
DATA_BLOCK DB3417
TITLE=
VERSION : 0.1

STRUCT
   CM_ID : STRING  [8 ] := '=PRM'; //COMPOSITE MACHINE
   STATION_ID : STRING  [8 ] := '++OP10'; //STATION - TRATTO - ZONE
   ELEMENT_ID : STRING  [8 ] := '+80FAN95'; //ELEMENT
   DB_ID : INT := 1 ; //DB SIZE OR TYPE
   PART_STYLE : STRING  [12 ]; //PART STYLE ON LAST STATION
   ACT_CYCLE_TIME : INT ; //ACTUAL CYCLE TIME FOR THIS STYLE
   COUNT_GOOD : INT ; //COUNTER GOOD PIECES
   COUNT_SCRAP : INT ; //COUNTER SCRAP PIECES
   SPARE_00 : ARRAY  [0 .. 15 ] OF //SPARE INTEGER
   INT ;
   SPARE_01 : ARRAY  [0 .. 17 ] OF //SPARE INTEGER
   INT ;
   CODE_EVENT : ARRAY  [0 .. 7 ] OF //CODE EVENT - EXTENDED FAULT CODE DIAGNOSTIC
   INT ;
   EVENT : STRUCT
E0000 : BOOL ; //+80FAN95-U1;MS.GENERALI ERRORE;1
E0001 : BOOL ; //+80FAN95-U1;MS.GENERALI AVVERTIMENTO;2
E0002 : BOOL ; //+80FAN95-U1;MS.MODALITA MANUALE;16
E0003 : BOOL ; //+80FAN95-U1;MS.MODO AUTOMATICO;19
E0004 : BOOL ; //+80FAN95-U1;MS.RILASCIO;17
E0005 : BOOL ; //+80FAN95-U1; MS. MOTORE ON;58
E0006 : BOOL ; //+80FAN95-U1; MS. MOTORE OFF;58
E0007 : BOOL ; //+80FAN95-U1; MS. MOTORE ON FRONTE POSITIVO;58
E0008 : BOOL ; //+80FAN95-U1; MS. FREQUENZA OK;58
E0009 : BOOL ; //+80FAN95-U1; MS. LOCALE DI CONTROLLO INTERRUTTORE ABILITATO;58
E0010 : BOOL ; //+80FAN95-U1; MS. ARRESTO A SUO AGIO;58
E0011 : BOOL ; //+80FAN95-U1; MS. LAST TASTO PREMUTO;58
E0012 : BOOL ; //+80FAN95-U1; MS. MS_14;58
E0013 : BOOL ; //+80FAN95-U1; MS. MS_15;58
E0014 : BOOL ; //+80FAN95-U1; MS. RES_WO_SAFETY_TEST;58
E0015 : BOOL ; //+80FAN95-U1; MS. MOTORE OFF FRONTE NEGATIVO;58
E0016 : BOOL ; //+80FAN95-U1;ME.MOTORE PROTEZIONE NON OK;1
E0017 : BOOL ; //+80FAN95-U1;ME.RUNTIME;1
E0018 : BOOL ; //+80FAN95-U1;ME.FREQUENZA CONVERTITORE PRONTO ERRORE;1
E0019 : BOOL ; //+80FAN95-U1;ME.FREQUENZA CONVERTITORE INTERNO ERRORE;1
E0020 : BOOL ; //+80FAN95-U1;ME.FREQUENZA CONVERTITORE DI VELOCITA ERRORE;1
E0021 : BOOL ; //+80FAN95-U1;ME.FREQUENZA CONVERTITORE MOTORE SOVRACCARICO;1
E0022 : BOOL ; //+80FAN95-U1; ME. FREQUENZA CONVERTITORE MOTORE SOVRACCARICO;58
E0023 : BOOL ; //+80FAN95-U1;ME.FREQUENZA CONVERTITORE AVVERTIMENTO;2
E0024 : BOOL ; //+80FAN95-U1; ME. FREQUENZA CONVERTITORE CORRENTE LIMITE DI ATTENZIONE;58
E0025 : BOOL ; //+80FAN95-U1;ME.PTC AVVERTIMENTO;2
E0026 : BOOL ; //+80FAN95-U1;ME.INTERRUTTORE PER MANUTENZIONE ERROR RILASCIO;1
E0027 : BOOL ; //+80FAN95-U1;ME.INTERRUTTORE PER MANUTENZIONE ERROR CORRENTE TAGLIARE;1
E0028 : BOOL ; //+80FAN95-U1; ME. ME_14;58
E0029 : BOOL ; //+80FAN95-U1; ME. ME_15;58
E0030 : BOOL ; //+80FAN95-U1; ME. ME_16;58
E0031 : BOOL ; //+80FAN95-U1; ME. ME_17;58
E0032 : BOOL ; //+80FAN95-B32F;MS.GENERALI ERRORE;1
E0033 : BOOL ; //+80FAN95-B32F;MS.GENERALI AVVERTIMENTO;2
E0034 : BOOL ; //+80FAN95-B32F; MS. MS_02;58
E0035 : BOOL ; //+80FAN95-B32F; MS. MS_03;58
E0036 : BOOL ; //+80FAN95-B32F; MS. MS_04;58
E0037 : BOOL ; //+80FAN95-B32F; MS. MS_05;58
E0038 : BOOL ; //+80FAN95-B32F; MS. MS_06;58
E0039 : BOOL ; //+80FAN95-B32F; MS. BINARIO OK;58
E0040 : BOOL ; //+80FAN95-B32F;MS.L03 MASSIMO AVVERTIMENTO;2
E0041 : BOOL ; //+80FAN95-B32F;MS.L02 MINIMO AVVERTIMENTO;2
E0042 : BOOL ; //+80FAN95-B32F; MS. MS_12;58
E0043 : BOOL ; //+80FAN95-B32F; MS. MS_13;58
E0044 : BOOL ; //+80FAN95-B32F; MS. MS_14;58
E0045 : BOOL ; //+80FAN95-B32F; MS. MS_15;58
E0046 : BOOL ; //+80FAN95-B32F; MS. MS_16;58
E0047 : BOOL ; //+80FAN95-B32F; MS. MS_17;58
E0048 : BOOL ; //+80FAN95-B32F;ME.L04 MASSIMO ERRORE;1
E0049 : BOOL ; //+80FAN95-B32F;ME.L01 MINIMO ERRORE;1
E0050 : BOOL ; //+80FAN95-B32F;ME.ALLARME;1
E0051 : BOOL ; //+80FAN95-B32F; ME. ME_03;58
E0052 : BOOL ; //+80FAN95-B32F; ME. ME_04;58
E0053 : BOOL ; //+80FAN95-B32F; ME. ME_05;58
E0054 : BOOL ; //+80FAN95-B32F; ME. ME_06;58
E0055 : BOOL ; //+80FAN95-B32F; ME. ME_07;58
E0056 : BOOL ; //+80FAN95-B32F;ME.L03 MASSIMO AVVERTIMENTO;2
E0057 : BOOL ; //+80FAN95-B32F;ME.L02 MINIMO AVVERTIMENTO;2
E0058 : BOOL ; //+80FAN95-B32F; ME. ME_12;58
E0059 : BOOL ; //+80FAN95-B32F; ME. ME_13;58
E0060 : BOOL ; //+80FAN95-B32F; ME. ME_14;58
E0061 : BOOL ; //+80FAN95-B32F; ME. ME_15;58
E0062 : BOOL ; //+80FAN95-B32F; ME. ME_16;58
E0063 : BOOL ; //+80FAN95-B32F; ME. ME_17;58

E0064 : BOOL ; //+80FAN95-B85; MS. ERRORE GENERALE;1
E0065 : BOOL ; //+80FAN95-B85;MS. PREALLARME;2
E0066 : BOOL ; //+80FAN95-B85;MS. ALLARME;1
E0067 : BOOL ; //+80FAN95-B85; MS. RES03;58
E0068 : BOOL ; //+80FAN95-B85; MS. RES04;58
E0069 : BOOL ; //+80FAN95-B85; MS. RES05;58
E0070 : BOOL ; //+80FAN95-B85; MS. RES06;58
E0071 : BOOL ; //+80FAN95-B85; MS. RES07;58
E0072 : BOOL ; //+80FAN95-B85; MS. RES10;58
E0073 : BOOL ; //+80FAN95-B85; MS. RES11;58
E0074 : BOOL ; //+80FAN95-B85; MS. RES12;58
E0075 : BOOL ; //+80FAN95-B85; MS. RES13;58
E0076 : BOOL ; //+80FAN95-B85; MS. RES14;58
E0077 : BOOL ; //+80FAN95-B85; MS. RES15;58
E0078 : BOOL ; //+80FAN95-B85; MS. RES16;58
E0079 : BOOL ; //+80FAN95-B85; MS. RES17;58
E0080 : BOOL ; //+80FAN95-B85;ME.PREALLARME;2
E0081 : BOOL ; //+80FAN95-B85;ME.ALLARME;1
E0082 : BOOL ; //+80FAN95-B85;ME.SENSORE GUASTO;1
E0083 : BOOL ; //+80FAN95-B85; ME. RES03;58
E0084 : BOOL ; //+80FAN95-B85; ME. RES04;58
E0085 : BOOL ; //+80FAN95-B85; ME. RES05;58
E0086 : BOOL ; //+80FAN95-B85; ME. RES06;58
E0087 : BOOL ; //+80FAN95-B85; ME. RES07;58
E0088 : BOOL ; //+80FAN95-B85; ME. RES10;58
E0089 : BOOL ; //+80FAN95-B85; ME. RES11;58
E0090 : BOOL ; //+80FAN95-B85; ME. RES12;58
E0091 : BOOL ; //+80FAN95-B85; ME. RES13;58
E0092 : BOOL ; //+80FAN95-B85; ME. RES14;58
E0093 : BOOL ; //+80FAN95-B85; ME. RES15;58
E0094 : BOOL ; //+80FAN95-B85; ME. RES16;58
E0095 : BOOL ; //+80FAN95-B85; ME. RES17;58
E0096 : BOOL ;
E0097 : BOOL ;
E0098 : BOOL ;
E0099 : BOOL ;
E0100 : BOOL ;
E0101 : BOOL ;
E0102 : BOOL ;
E0103 : BOOL ;
E0104 : BOOL ;
E0105 : BOOL ;
E0106 : BOOL ;
E0107 : BOOL ;
E0108 : BOOL ;
E0109 : BOOL ;
E0110 : BOOL ;
E0111 : BOOL ;
E0112 : BOOL ;
E0113 : BOOL ;
E0114 : BOOL ;
E0115 : BOOL ;
E0116 : BOOL ;
E0117 : BOOL ;
E0118 : BOOL ;
E0119 : BOOL ;
E0120 : BOOL ;
E0121 : BOOL ;
E0122 : BOOL ;
E0123 : BOOL ;
E0124 : BOOL ;
E0125 : BOOL ;
E0126 : BOOL ;
E0127 : BOOL ;
E0128 : BOOL ;
E0129 : BOOL ;
E0130 : BOOL ;
E0131 : BOOL ;
E0132 : BOOL ;
E0133 : BOOL ;
E0134 : BOOL ;
E0135 : BOOL ;
E0136 : BOOL ;
E0137 : BOOL ;
E0138 : BOOL ;
E0139 : BOOL ;
E0140 : BOOL ;
E0141 : BOOL ;
E0142 : BOOL ;
E0143 : BOOL ;
E0144 : BOOL ;
E0145 : BOOL ;
E0146 : BOOL ;
E0147 : BOOL ;
E0148 : BOOL ;
E0149 : BOOL ;
E0150 : BOOL ;
E0151 : BOOL ;
E0152 : BOOL ;
E0153 : BOOL ;
E0154 : BOOL ;
E0155 : BOOL ;
E0156 : BOOL ;
E0157 : BOOL ;
E0158 : BOOL ;
E0159 : BOOL ;
E0160 : BOOL ;
E0161 : BOOL ;
E0162 : BOOL ;
E0163 : BOOL ;
E0164 : BOOL ;
E0165 : BOOL ;
E0166 : BOOL ;
E0167 : BOOL ;
E0168 : BOOL ;
E0169 : BOOL ;
E0170 : BOOL ;
E0171 : BOOL ;
E0172 : BOOL ;
E0173 : BOOL ;
E0174 : BOOL ;
E0175 : BOOL ;
E0176 : BOOL ;
E0177 : BOOL ;
E0178 : BOOL ;
E0179 : BOOL ;
E0180 : BOOL ;
E0181 : BOOL ;
E0182 : BOOL ;
E0183 : BOOL ;
E0184 : BOOL ;
E0185 : BOOL ;
E0186 : BOOL ;
E0187 : BOOL ;
E0188 : BOOL ;
E0189 : BOOL ;
E0190 : BOOL ;
E0191 : BOOL ;
E0192 : BOOL ;
E0193 : BOOL ;
E0194 : BOOL ;
E0195 : BOOL ;
E0196 : BOOL ;
E0197 : BOOL ;
E0198 : BOOL ;
E0199 : BOOL ;
E0200 : BOOL ;
E0201 : BOOL ;
E0202 : BOOL ;
E0203 : BOOL ;
E0204 : BOOL ;
E0205 : BOOL ;
E0206 : BOOL ;
E0207 : BOOL ;
E0208 : BOOL ;
E0209 : BOOL ;
E0210 : BOOL ;
E0211 : BOOL ;
E0212 : BOOL ;
E0213 : BOOL ;
E0214 : BOOL ;
E0215 : BOOL ;
E0216 : BOOL ;
E0217 : BOOL ;
E0218 : BOOL ;
E0219 : BOOL ;
E0220 : BOOL ;
E0221 : BOOL ;
E0222 : BOOL ;
E0223 : BOOL ;
E0224 : BOOL ;
E0225 : BOOL ;
E0226 : BOOL ;
E0227 : BOOL ;
E0228 : BOOL ;
E0229 : BOOL ;
E0230 : BOOL ;
E0231 : BOOL ;
E0232 : BOOL ;
E0233 : BOOL ;
E0234 : BOOL ;
E0235 : BOOL ;
E0236 : BOOL ;
E0237 : BOOL ;
E0238 : BOOL ;
E0239 : BOOL ;
E0240 : BOOL ;
E0241 : BOOL ;
E0242 : BOOL ;
E0243 : BOOL ;
E0244 : BOOL ;
E0245 : BOOL ;
E0246 : BOOL ;
E0247 : BOOL ;
E0248 : BOOL ;
E0249 : BOOL ;
E0250 : BOOL ;
E0251 : BOOL ;
E0252 : BOOL ;
E0253 : BOOL ;
E0254 : BOOL ;
E0255 : BOOL ;
END_STRUCT;
END_STRUCT;
BEGIN
CM_ID := '=PRM';
STATION_ID := '++OP10';
ELEMENT_ID := '+80FAN95';
DB_ID := 1 ;
PART_STYLE := '';
ACT_CYCLE_TIME := 0;
COUNT_GOOD := 0;
COUNT_SCRAP := 0;
SPARE_00[0] := 0;
SPARE_00[1] := 0;
SPARE_00[2] := 0;
SPARE_00[3] := 0;
SPARE_00[4] := 0;
SPARE_00[5] := 0;
SPARE_00[6] := 0;
SPARE_00[7] := 0;
SPARE_00[8] := 0;
SPARE_00[9] := 0;
SPARE_00[10] := 0;
SPARE_00[11] := 0;
SPARE_00[12] := 0;
SPARE_00[13] := 0;
SPARE_00[14] := 0;
SPARE_00[15] := 0;
SPARE_01[0] := 0;
SPARE_01[1] := 0;
SPARE_01[2] := 0;
SPARE_01[3] := 0;
SPARE_01[4] := 0;
SPARE_01[5] := 0;
SPARE_01[6] := 0;
SPARE_01[7] := 0;
SPARE_01[8] := 0;
SPARE_01[9] := 0;
SPARE_01[10] := 0;
SPARE_01[11] := 0;
SPARE_01[12] := 0;
SPARE_01[13] := 0;
SPARE_01[14] := 0;
SPARE_01[15] := 0;
SPARE_01[16] := 0;
SPARE_01[17] := 0;
CODE_EVENT[0] := 0;
CODE_EVENT[1] := 0;
CODE_EVENT[2] := 0;
CODE_EVENT[3] := 0;
CODE_EVENT[4] := 0;
CODE_EVENT[5] := 0;
CODE_EVENT[6] := 0;
CODE_EVENT[7] := 0;
EVENT.E0000 := FALSE;
EVENT.E0001 := FALSE;
EVENT.E0002 := FALSE;
EVENT.E0003 := FALSE;
EVENT.E0004 := FALSE;
EVENT.E0005 := FALSE;
EVENT.E0006 := FALSE;
EVENT.E0007 := FALSE;
EVENT.E0008 := FALSE;
EVENT.E0009 := FALSE;
EVENT.E0010 := FALSE;
EVENT.E0011 := FALSE;
EVENT.E0012 := FALSE;
EVENT.E0013 := FALSE;
EVENT.E0014 := FALSE;
EVENT.E0015 := FALSE;
EVENT.E0016 := FALSE;
EVENT.E0017 := FALSE;
EVENT.E0018 := FALSE;
EVENT.E0019 := FALSE;
EVENT.E0020 := FALSE;
EVENT.E0021 := FALSE;
EVENT.E0022 := FALSE;
EVENT.E0023 := FALSE;
EVENT.E0024 := FALSE;
EVENT.E0025 := FALSE;
EVENT.E0026 := FALSE;
EVENT.E0027 := FALSE;
EVENT.E0028 := FALSE;
EVENT.E0029 := FALSE;
EVENT.E0030 := FALSE;
EVENT.E0031 := FALSE;
EVENT.E0032 := FALSE;
EVENT.E0033 := FALSE;
EVENT.E0034 := FALSE;
EVENT.E0035 := FALSE;
EVENT.E0036 := FALSE;
EVENT.E0037 := FALSE;
EVENT.E0038 := FALSE;
EVENT.E0039 := FALSE;
EVENT.E0040 := FALSE;
EVENT.E0041 := FALSE;
EVENT.E0042 := FALSE;
EVENT.E0043 := FALSE;
EVENT.E0044 := FALSE;
EVENT.E0045 := FALSE;
EVENT.E0046 := FALSE;
EVENT.E0047 := FALSE;
EVENT.E0048 := FALSE;
EVENT.E0049 := FALSE;
EVENT.E0050 := FALSE;
EVENT.E0051 := FALSE;
EVENT.E0052 := FALSE;
EVENT.E0053 := FALSE;
EVENT.E0054 := FALSE;
EVENT.E0055 := FALSE;
EVENT.E0056 := FALSE;
EVENT.E0057 := FALSE;
EVENT.E0058 := FALSE;
EVENT.E0059 := FALSE;
EVENT.E0060 := FALSE;
EVENT.E0061 := FALSE;
EVENT.E0062 := FALSE;
EVENT.E0063 := FALSE;
EVENT.E0064 := FALSE;
EVENT.E0065 := FALSE;
EVENT.E0066 := FALSE;
EVENT.E0067 := FALSE;
EVENT.E0068 := FALSE;
EVENT.E0069 := FALSE;
EVENT.E0070 := FALSE;
EVENT.E0071 := FALSE;
EVENT.E0072 := FALSE;
EVENT.E0073 := FALSE;
EVENT.E0074 := FALSE;
EVENT.E0075 := FALSE;
EVENT.E0076 := FALSE;
EVENT.E0077 := FALSE;
EVENT.E0078 := FALSE;
EVENT.E0079 := FALSE;
EVENT.E0080 := FALSE;
EVENT.E0081 := FALSE;
EVENT.E0082 := FALSE;
EVENT.E0083 := FALSE;
EVENT.E0084 := FALSE;
EVENT.E0085 := FALSE;
EVENT.E0086 := FALSE;
EVENT.E0087 := FALSE;
EVENT.E0088 := FALSE;
EVENT.E0089 := FALSE;
EVENT.E0090 := FALSE;
EVENT.E0091 := FALSE;
EVENT.E0092 := FALSE;
EVENT.E0093 := FALSE;
EVENT.E0094 := FALSE;
EVENT.E0095 := FALSE;
EVENT.E0096 := FALSE;
EVENT.E0097 := FALSE;
EVENT.E0098 := FALSE;
EVENT.E0099 := FALSE;
EVENT.E0100 := FALSE;
EVENT.E0101 := FALSE;
EVENT.E0102 := FALSE;
EVENT.E0103 := FALSE;
EVENT.E0104 := FALSE;
EVENT.E0105 := FALSE;
EVENT.E0106 := FALSE;
EVENT.E0107 := FALSE;
EVENT.E0108 := FALSE;
EVENT.E0109 := FALSE;
EVENT.E0110 := FALSE;
EVENT.E0111 := FALSE;
EVENT.E0112 := FALSE;
EVENT.E0113 := FALSE;
EVENT.E0114 := FALSE;
EVENT.E0115 := FALSE;
EVENT.E0116 := FALSE;
EVENT.E0117 := FALSE;
EVENT.E0118 := FALSE;
EVENT.E0119 := FALSE;
EVENT.E0120 := FALSE;
EVENT.E0121 := FALSE;
EVENT.E0122 := FALSE;
EVENT.E0123 := FALSE;
EVENT.E0124 := FALSE;
EVENT.E0125 := FALSE;
EVENT.E0126 := FALSE;
EVENT.E0127 := FALSE;
EVENT.E0128 := FALSE;
EVENT.E0129 := FALSE;
EVENT.E0130 := FALSE;
EVENT.E0131 := FALSE;
EVENT.E0132 := FALSE;
EVENT.E0133 := FALSE;
EVENT.E0134 := FALSE;
EVENT.E0135 := FALSE;
EVENT.E0136 := FALSE;
EVENT.E0137 := FALSE;
EVENT.E0138 := FALSE;
EVENT.E0139 := FALSE;
EVENT.E0140 := FALSE;
EVENT.E0141 := FALSE;
EVENT.E0142 := FALSE;
EVENT.E0143 := FALSE;
EVENT.E0144 := FALSE;
EVENT.E0145 := FALSE;
EVENT.E0146 := FALSE;
EVENT.E0147 := FALSE;
EVENT.E0148 := FALSE;
EVENT.E0149 := FALSE;
EVENT.E0150 := FALSE;
EVENT.E0151 := FALSE;
EVENT.E0152 := FALSE;
EVENT.E0153 := FALSE;
EVENT.E0154 := FALSE;
EVENT.E0155 := FALSE;
EVENT.E0156 := FALSE;
EVENT.E0157 := FALSE;
EVENT.E0158 := FALSE;
EVENT.E0159 := FALSE;
EVENT.E0160 := FALSE;
EVENT.E0161 := FALSE;
EVENT.E0162 := FALSE;
EVENT.E0163 := FALSE;
EVENT.E0164 := FALSE;
EVENT.E0165 := FALSE;
EVENT.E0166 := FALSE;
EVENT.E0167 := FALSE;
EVENT.E0168 := FALSE;
EVENT.E0169 := FALSE;
EVENT.E0170 := FALSE;
EVENT.E0171 := FALSE;
EVENT.E0172 := FALSE;
EVENT.E0173 := FALSE;
EVENT.E0174 := FALSE;
EVENT.E0175 := FALSE;
EVENT.E0176 := FALSE;
EVENT.E0177 := FALSE;
EVENT.E0178 := FALSE;
EVENT.E0179 := FALSE;
EVENT.E0180 := FALSE;
EVENT.E0181 := FALSE;
EVENT.E0182 := FALSE;
EVENT.E0183 := FALSE;
EVENT.E0184 := FALSE;
EVENT.E0185 := FALSE;
EVENT.E0186 := FALSE;
EVENT.E0187 := FALSE;
EVENT.E0188 := FALSE;
EVENT.E0189 := FALSE;
EVENT.E0190 := FALSE;
EVENT.E0191 := FALSE;
EVENT.E0192 := FALSE;
EVENT.E0193 := FALSE;
EVENT.E0194 := FALSE;
EVENT.E0195 := FALSE;
EVENT.E0196 := FALSE;
EVENT.E0197 := FALSE;
EVENT.E0198 := FALSE;
EVENT.E0199 := FALSE;
EVENT.E0200 := FALSE;
EVENT.E0201 := FALSE;
EVENT.E0202 := FALSE;
EVENT.E0203 := FALSE;
EVENT.E0204 := FALSE;
EVENT.E0205 := FALSE;
EVENT.E0206 := FALSE;
EVENT.E0207 := FALSE;
EVENT.E0208 := FALSE;
EVENT.E0209 := FALSE;
EVENT.E0210 := FALSE;
EVENT.E0211 := FALSE;
EVENT.E0212 := FALSE;
EVENT.E0213 := FALSE;
EVENT.E0214 := FALSE;
EVENT.E0215 := FALSE;
EVENT.E0216 := FALSE;
EVENT.E0217 := FALSE;
EVENT.E0218 := FALSE;
EVENT.E0219 := FALSE;
EVENT.E0220 := FALSE;
EVENT.E0221 := FALSE;
EVENT.E0222 := FALSE;
EVENT.E0223 := FALSE;
EVENT.E0224 := FALSE;
EVENT.E0225 := FALSE;
EVENT.E0226 := FALSE;
EVENT.E0227 := FALSE;
EVENT.E0228 := FALSE;
EVENT.E0229 := FALSE;
EVENT.E0230 := FALSE;
EVENT.E0231 := FALSE;
EVENT.E0232 := FALSE;
EVENT.E0233 := FALSE;
EVENT.E0234 := FALSE;
EVENT.E0235 := FALSE;
EVENT.E0236 := FALSE;
EVENT.E0237 := FALSE;
EVENT.E0238 := FALSE;
EVENT.E0239 := FALSE;
EVENT.E0240 := FALSE;
EVENT.E0241 := FALSE;
EVENT.E0242 := FALSE;
EVENT.E0243 := FALSE;
EVENT.E0244 := FALSE;
EVENT.E0245 := FALSE;
EVENT.E0246 := FALSE;
EVENT.E0247 := FALSE;
EVENT.E0248 := FALSE;
EVENT.E0249 := FALSE;
EVENT.E0250 := FALSE;
EVENT.E0251 := FALSE;
EVENT.E0252 := FALSE;
EVENT.E0253 := FALSE;
EVENT.E0254 := FALSE;
EVENT.E0255 := FALSE;
END_DATA_BLOCK
